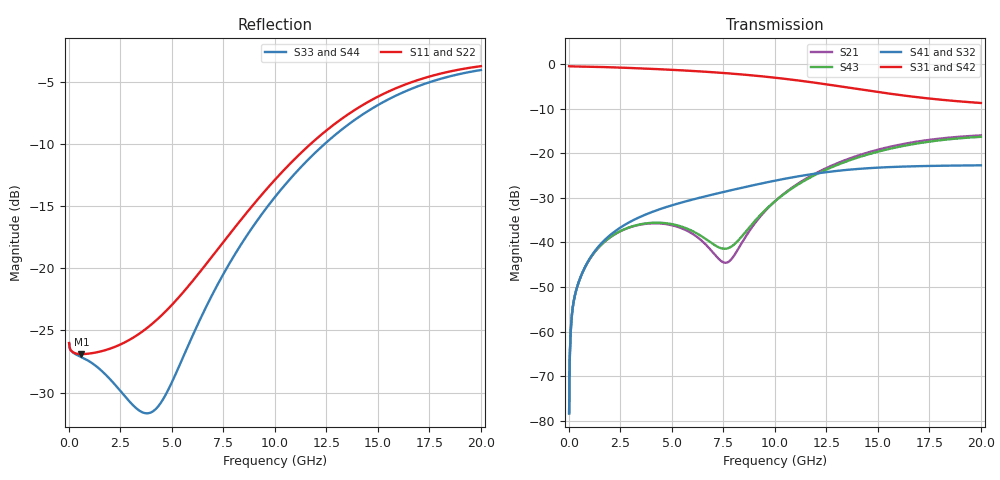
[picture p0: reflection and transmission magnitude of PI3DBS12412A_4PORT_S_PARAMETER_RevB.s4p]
! NPort=4 DATA=2000 NOISE=0 GROUPDELAY=0 COMPLEX_DATAFORMAT=POLAR
! NumOfBlock=1 NumOfParam=0
! .MODEL Smodel S TSTONEFILE=PI3DBS12412A_4PORT_S_PARAMETER_RevB.s4p TYPE=S
!  -- The above .MODEL line can be used for the S element in the netlist.
!PORT1 = INPUT+
!PORT2 = INPUT-
!PORT3 = OUTPUT+
!PORT4 = OUTPUT-
# Hz S MA R  50
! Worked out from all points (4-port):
!   2000 points, 10 MHz to 20 GHz, reference 50 ohm
!   strongest paths, dB at 10 MHz, 5.01 GHz, 10.01 GHz, 15.01 GHz, 20 GHz:
!     S31: -0.5, -1.3, -3.0, -6.3, -8.7
!     S42: -0.5, -1.3, -3.1, -6.3, -8.7
!     S41: -78.4, -31.7, -26.1, -23.2, -22.7
!     S32: -78.4, -31.7, -26.1, -23.2, -22.7
!     S43: -78.3, -35.9, -30.7, -19.6, -16.3
!     S21: -78.3, -36.2, -30.8, -19.2, -16.0
!   lowest |S11| = -26.9 dB at 610 MHz (marker M1), VSWR 1.09, Z = 54.2 - j2.18 ohm
!   |S11| at or under -10 dB: start of sweep to 11.75 GHz
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1e7  0.05001 -2.1  0.0001212 88.4  0.9486 -0.2  0.0001209 88.4
     0.0001212 88.4  0.05001 -2.1  0.0001209 88.4  0.9486 -0.2
     0.9486 -0.2  0.0001209 88.4  0.05002 -2.0  0.0001212 88.4
     0.0001209 88.4  0.9486 -0.2  0.0001212 88.4  0.05002 -2.0
1.9e8  0.04601 -9.9  0.00189 71.0  0.9427 -2.3  0.001886 70.8
       0.00189 71.0  0.04601 -9.9  0.001886 70.8  0.9427 -2.3
       0.9427 -2.3  0.001886 70.8  0.04591 -7.8  0.00189 71.0
       0.001886 70.8  0.9427 -2.3  0.00189 71.0  0.04592 -7.8
6.1e8  0.04516 -26.5  0.004319 67.9  0.9394 -6.8  0.004328 67.5
       0.004319 67.9  0.04517 -26.5  0.004328 67.5  0.9394 -6.8
       0.9394 -6.8  0.004328 67.5  0.04393 -19.8  0.004317 68.2
       0.004328 67.5  0.9394 -6.8  0.004317 68.2  0.04393 -19.8
3.85e9  0.05799 -143.9  0.01626 46.1  0.8885 -41.1  0.02111 44.3
        0.01626 46.1  0.05821 -144.1  0.02111 44.3  0.8884 -41.1
        0.8883 -41.2  0.0211 44.3  0.02613 -141.9  0.01646 48.6
        0.02111 44.3  0.8881 -41.2  0.01646 48.6  0.02631 -142.1
7.59e9  0.1302 117.3  0.005905 82.0  0.7931 -79.5  0.03719 15.2
        0.005905 82.0  0.1305 117.3  0.03719 15.2  0.7928 -79.5
        0.7928 -79.6  0.03717 15.1  0.09767 94.2  0.008483 80.4
        0.03717 15.1  0.7925 -79.6  0.008483 80.4  0.09787 94.3
1.221e10  0.3416 40.6  0.06345 123.3  0.6069 -125.0  0.06021 -27.2
          0.06345 123.3  0.3419 40.6  0.06021 -27.2  0.6066 -125.0
          0.6065 -125.1  0.06018 -27.3  0.3045 31.3  0.06115 117.9
          0.06018 -27.3  0.6062 -125.1  0.06115 117.9  0.3047 31.3
2e10  0.6481 -40.6  0.1586 60.0  0.3669 -179.2  0.07332 -106.3
      0.1586 60.0  0.6483 -40.6  0.07332 -106.3  0.3667 -179.2
      0.3665 -179.4  0.07324 -106.5  0.6255 -42.2  0.1529 59.6
      0.07324 -106.5  0.3663 -179.4  0.1529 59.6  0.6257 -42.2
